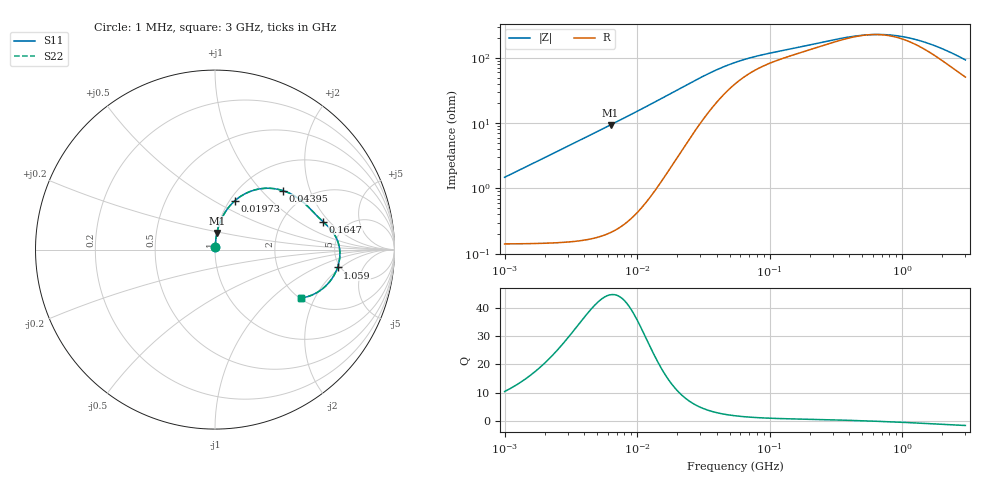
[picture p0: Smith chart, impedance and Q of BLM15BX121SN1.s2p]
! BLM15BX121SN1
# Hz S RI R 50
!Freq.(Hz) S11(Real) S11(Imag) S21(Real) S21(Imag) S12(Real) S12(Imag) S22(Real) S22(Imag)
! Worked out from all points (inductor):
!   401 points, 1 MHz to 3 GHz, reference 50 ohm
!   read as one part in series: L = 235 nH near 1.041 MHz
!   highest Q = 44.6 at 6.306 MHz (marker M1), where L = 237 nH
!   self-resonance near 589.8 MHz
!   S11 on the Smith chart (normalised r, x): 1 MHz: 1.00, +0.03; 19.73 MHz: 1.06, +0.63; 43.95 MHz: 1.52, +1.33; 164.7 MHz: 3.35, +1.70; 1.059 GHz: 4.74, -1.80; 3 GHz: 2.02, -1.56
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1000000  0.00162 0.0147  0.9984 -0.0147  0.9984 -0.0147  0.00162 0.0147
3823119  0.00476 0.0562  0.9952 -0.0562  0.9952 -0.0562  0.00476 0.0562
6305767  0.0108 0.0928  0.9892 -0.0928  0.9892 -0.0928  0.0108 0.0928
9794439  0.0253 0.1441  0.9747 -0.1441  0.9747 -0.1441  0.0253 0.1441
1.461624e7  0.0587 0.2116  0.9413 -0.2116  0.9413 -0.2116  0.0587 0.2116
1.973457e7  0.1108 0.2723  0.8892 -0.2723  0.8892 -0.2723  0.1108 0.2723
2.41077e7  0.1646 0.3097  0.8354 -0.3097  0.8354 -0.3097  0.1646 0.3097
3.00453e7  0.2403 0.3367  0.7597 -0.3367  0.7597 -0.3367  0.2403 0.3367
3.597591e7  0.3085 0.3415  0.6915 -0.3415  0.6915 -0.3415  0.3085 0.3415
4.394807e7  0.3802 0.328  0.6198 -0.328  0.6198 -0.328  0.3802 0.328
5.477226e7  0.445 0.298  0.555 -0.298  0.555 -0.298  0.445 0.298
8.338914e7  0.5253 0.2324  0.4747 -0.2324  0.4747 -0.2324  0.5253 0.2324
1.646891e8  0.6014 0.1562  0.3986 -0.1562  0.3986 -0.1562  0.6014 0.1562
2.094008e8  0.6255 0.1333  0.3745 -0.1333  0.3745 -0.1333  0.6255 0.1333
4.66327e8  0.6874 0.0354  0.3126 -0.0354  0.3126 -0.0354  0.6874 0.0354
6.171487e8  0.6952 -0.00714  0.3048 0.00714  0.3048 0.00714  0.6952 -0.00714
8.005644e8  0.6943 -0.0499  0.3057 0.0499  0.3057 0.0499  0.6943 -0.0499
1.059487e9  0.6829 -0.0995  0.3171 0.0995  0.3171 0.0995  0.6829 -0.0995
1.402151e9  0.6576 -0.1526  0.3424 0.1526  0.3424 0.1526  0.6576 -0.1526
1.818868e9  0.6168 -0.2027  0.3832 0.2027  0.3832 0.2027  0.6168 -0.2027
2.407135e9  0.5487 -0.2495  0.4513 0.2495  0.4513 0.2495  0.5487 -0.2495
3e9  0.4767 -0.2707  0.5233 0.2707  0.5233 0.2707  0.4767 -0.2707
